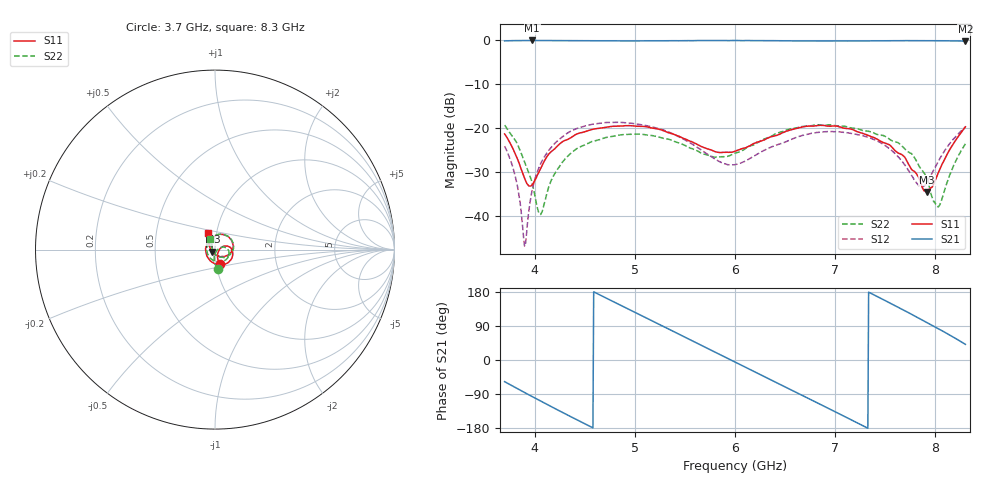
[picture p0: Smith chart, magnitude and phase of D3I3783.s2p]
! 4/13/2021 4:20:18 PM
! C:\USERS\DITOM\DESKTOP\SINGLE JUNCTION ISOLATOR DATA\3.7-8.3 GHZ (D3I3783).S2P
! CHANNEL.1
! TR.MEASUREMENT
! CORRECTED.DATA
# GHZ S RI R 50.0
! FREQ.GHZ  S11RE  S11IM  S21RE  S21IM  S12RE  S12IM  S22RE  S22IM
!; PortSelection: Port_12
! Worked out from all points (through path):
!   601 points, 3.7 GHz to 8.3 GHz, reference 50 ohm
!   highest |S21| = -0.17 dB at 3.976 GHz (marker M1); lowest = -0.3 dB at 8.3 GHz (marker M2)
!   lowest |S11| = -34.6 dB at 7.917 GHz (marker M3), VSWR 1.04, Z = 48.6 - j1.17 ohm
!   |S11| at or under -10 dB: start of sweep to end of sweep
!   |S22| runs from -39.8 to -19.3 dB; largest |S21 - S12| = 1
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3.7  0.0266 -0.0804  0.5256 -0.8145  -0.0528 0.0317  0.0146 -0.1056
3.815  0.0145 -0.0455  0.2719 -0.9375  -0.0129 0.0218  -0.00302 -0.0691
3.899333  0.0151 -0.0217  0.0712 -0.976  0.00369 0.00256  -0.00442 -0.0403
3.976  0.0222 -0.00374  -0.1154 -0.9734  0.00763 -0.0181  0.00029 -0.023
4.060333  0.033 0.00971  -0.3106 -0.9285  0.000505 -0.039  0.00925 -0.00447
4.206  0.0548 0.0196  -0.6084 -0.7637  -0.0319 -0.0589  0.0288 0.0105
4.466667  0.0868 0.0113  -0.9351 -0.2736  -0.0991 -0.022  0.0603 0.0109
4.811667  0.0986 -0.0328  -0.8446 0.4765  -0.0774 0.0848  0.0786 -0.0194
5.026333  0.0814 -0.0642  -0.5178 0.8196  -0.0127 0.1089  0.0701 -0.047
5.241  0.0439 -0.0852  -0.0734 0.9691  0.045 0.0867  0.0411 -0.0663
5.586  -0.0264 -0.0623  0.6377 0.7379  0.0615 0.016  -0.0215 -0.0526
5.785333  -0.0488 -0.0236  0.9009 0.3792  0.045 -0.000326  -0.0425 -0.0184
6  -0.0481 0.0241  0.9752 -0.0908  0.0379 0.00109  -0.0445 0.0252
6.199333  -0.0266 0.0613  0.8311 -0.51  0.048 -0.002  -0.0237 0.0601
6.406333  0.011 0.0804  0.5018 -0.8326  0.0577 -0.0252  0.0139 0.084
6.766667  0.0825 0.0633  -0.2665 -0.9308  0.023 -0.0832  0.0853 0.0621
7.180667  0.0937 -0.0103  -0.9131 -0.3215  -0.0719 -0.0459  0.0984 -0.00613
7.541  0.0501 -0.0397  -0.8524 0.4699  -0.0429 0.0387  0.0627 -0.0392
7.832333  -1.61e-05 -0.0275  -0.3473 0.9122  0.0196 0.0101  0.0158 -0.0341
7.916667  -0.0142 -0.012  -0.1514 0.9644  0.0197 -0.0132  0.00297 -0.0261
8.031667  -0.0285 0.0126  0.1273 0.9648  -0.00183 -0.0418  -0.0118 -0.00434
8.3  -0.0403 0.0939  0.7222 0.6344  -0.1013 -0.00254  -0.0284 0.0589
